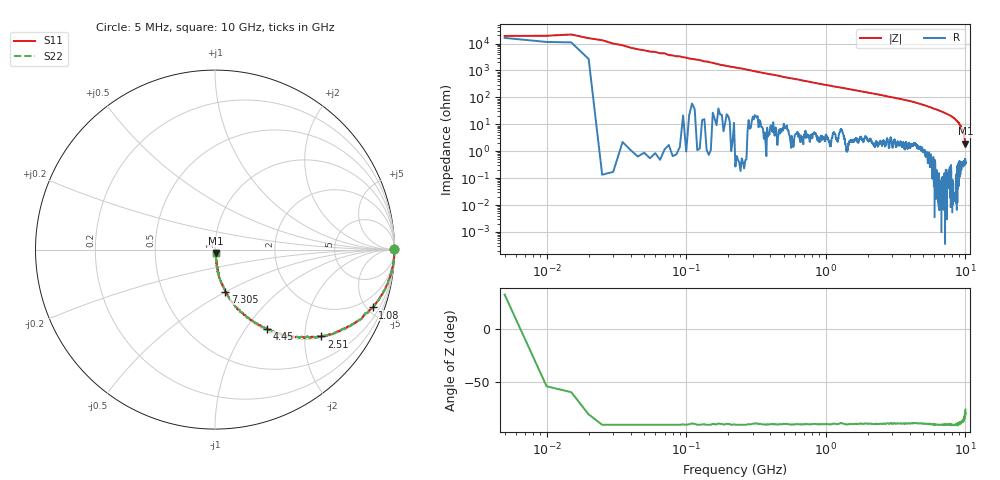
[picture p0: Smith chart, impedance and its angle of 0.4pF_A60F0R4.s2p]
! Amotech Co.,Ltd.
! http://www.amotech.co.kr/
! Part Number: A60F0R4
! These Parameters are Measured in Series Mode Connection
! Operation Temp=25[degC], DC Bias Voltage=0[V]
! Freq. Start=5[MHz] Stop=10[GHz], 2000[Steps]
! Date: Monday, July 20, 2020, 03:10:14
# GHZ S RI R 50.000000
!Freq.(Hz) S11(Real) S11(Imag) S21(Real) S21(Imag) S12(Real) S12(Imag) S22(Real) S22(Imag)
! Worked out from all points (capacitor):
!   2000 points, 5 MHz to 10 GHz, reference 50 ohm
!   read as one part in series: C = 544 fF near 55 MHz
!   lowest |Z| = 1.9 ohm at 10 GHz (marker M1)
!   S11 on the Smith chart (normalised r, x): 5 MHz: open; 1.08 GHz: 1.04, -5.44; 2.51 GHz: 1.04, -2.42; 4.45 GHz: 1.03, -1.26; 7.305 GHz: 1.00, -0.50; 10 GHz: 1.01, -0.04
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0.005  0.9956 0.00275  0.00441 -0.00275  0.00441 -0.00275  0.9956 0.00275
0.04  0.9998 -0.0143  0.000206 0.0143  0.000206 0.0143  0.9998 -0.0143
0.08  0.9992 -0.0276  0.000769 0.0276  0.000769 0.0276  0.9992 -0.0276
0.115  0.998 -0.0386  0.00204 0.0386  0.00204 0.0386  0.998 -0.0386
0.185  0.9957 -0.064  0.00434 0.064  0.00434 0.064  0.9957 -0.064
0.28  0.9894 -0.0955  0.0106 0.0955  0.0106 0.0955  0.9894 -0.0955
0.38  0.9816 -0.1297  0.0184 0.1297  0.0184 0.1297  0.9816 -0.1297
0.555  0.9634 -0.1851  0.0366 0.1851  0.0366 0.1851  0.9634 -0.1851
0.795  0.9273 -0.2545  0.0727 0.2545  0.0727 0.2545  0.9273 -0.2545
1.08  0.8792 -0.3225  0.1208 0.3225  0.1208 0.3225  0.8792 -0.3225
1.675  0.7617 -0.4198  0.2383 0.4198  0.2383 0.4198  0.7617 -0.4198
2.51  0.5926 -0.4838  0.4074 0.4838  0.4074 0.4838  0.5926 -0.4838
3.34  0.4447 -0.4873  0.5553 0.4873  0.5553 0.4873  0.4447 -0.4873
4.45  0.291 -0.4407  0.709 0.4407  0.709 0.4407  0.291 -0.4407
5.005  0.22 -0.4056  0.78 0.4056  0.78 0.4056  0.22 -0.4056
6.67  0.0861 -0.28  0.9139 0.28  0.9139 0.28  0.0861 -0.28
7.305  0.0583 -0.2342  0.9417 0.2342  0.9417 0.2342  0.0583 -0.2342
8.335  0.0255 -0.1601  0.9745 0.1601  0.9745 0.1601  0.0255 -0.1601
8.885  0.0169 -0.116  0.9831 0.116  0.9831 0.116  0.0169 -0.116
9.405  0.00878 -0.0717  0.9912 0.0717  0.9912 0.0717  0.00878 -0.0717
9.785  0.00497 -0.0378  0.995 0.0378  0.995 0.0378  0.00497 -0.0378
10  0.00495 -0.0182  0.9951 0.0182  0.9951 0.0182  0.00495 -0.0182
